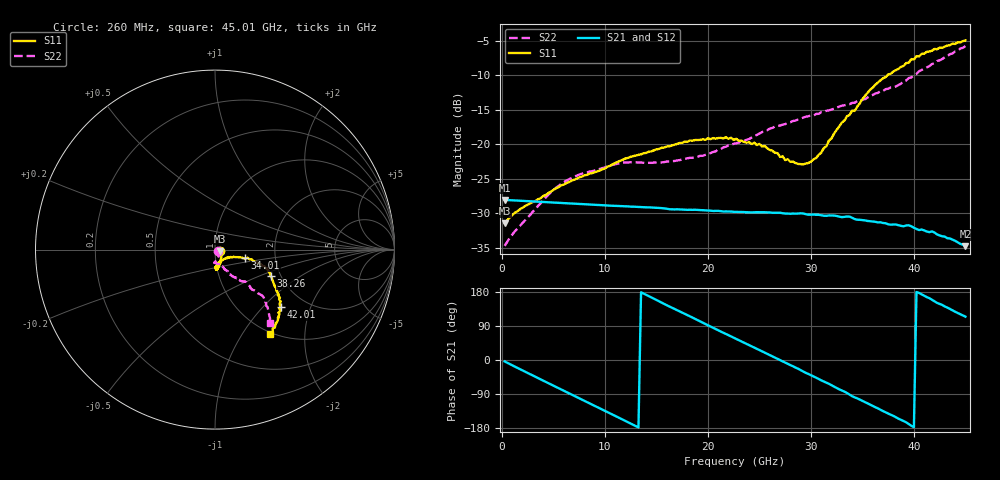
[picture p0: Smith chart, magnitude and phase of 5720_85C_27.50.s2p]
! Device:  ADRF5720
! Description: 0.5dB LSB GaAs MMIC 6-bit Digital Attenuator
! Frequency:  0.000009 -  40 GHz
! Ports:
!	RF1	= Port 1
!	RF2	= Port 2
! Vdd:  3.3 Volt
! Vss:  -3.3 Volt
! Control:  0/3.3 Volt
! State:  27.50 dB attenuation
! Data:  The device was measured using G-S-G Probes on a matrix board.
!  Data was collected using an calibrated 4 port network analyzer.
!  The reference plane for this measurement is at the launchers.
! Note:  Analog Devices supplies this data as a sample of measured data
!  for this product.  Your particular data for this product may vary.
!  Data was taken at 85 degrees C.
!  Analog Devices reserves the right to change this data at anytime.
# GHZ S DB R 45.0
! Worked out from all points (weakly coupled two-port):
!   180 points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, 260 MHz to 45.01 GHz, reference 45 ohm
!   highest |S21| = -28.07 dB at 260 MHz (marker M1); lowest = -34.8 dB at 45.01 GHz (marker M2)
!   lowest |S11| = -31.5 dB at 260 MHz (marker M3), VSWR 1.05, Z = 47.3 - j0.764 ohm
!   |S11| at or under -10 dB: start of sweep to 37.46 GHz
!   |S22| runs from -34.7 to -5.8 dB; largest |S21 - S12| = 0.00027
!   S11 on the Smith chart (normalised r, x): 260 MHz: 1.05, -0.02; 34.01 GHz: 1.40, -0.14; 38.26 GHz: 1.77, -0.59; 42.01 GHz: 1.52, -1.28; 45.01 GHz: 0.97, -1.34
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0.26  -31.47 -17.6  -28.07 -3.7  -28.06 -3.7  -34.73 -26.4
1.26  -29.93 -3.5  -28.15 -17.6  -28.14 -17.5  -32.61 -13.7
4.76  -26.87 -37.6  -28.43 -64.5  -28.41 -64.5  -26.96 -65.6
6.26  -25.63 -46.4  -28.55 -84.5  -28.53 -84.4  -25.28 -75.1
7.76  -24.72 -53.3  -28.67 -104.4  -28.66 -104.4  -24.28 -81.6
11.51  -22.39 -67.5  -28.97 -154.4  -28.96 -154.3  -22.72 -92.2
15.26  -20.69 -75.5  -29.24 154.8  -29.22 154.9  -22.64 -90.0
18.26  -19.46 -81.1  -29.50 115.2  -29.49 115.4  -21.98 -81.7
22.76  -19.22 -86.7  -29.80 55.5  -29.78 55.7  -19.87 -67.5
25.51  -20.24 -85.5  -29.86 19.6  -29.84 19.8  -18.05 -63.7
27.51  -22.31 -78.3  -30.05 -7.0  -30.03 -6.7  -17.10 -59.6
28.76  -22.87 -61.7  -30.05 -23.0  -30.02 -22.7  -16.44 -59.9
30.26  -22.21 -41.2  -30.19 -43.2  -30.17 -43.0  -15.86 -58.7
31.51  -20.31 -24.8  -30.38 -59.7  -30.37 -59.4  -15.17 -57.2
34.01  -15.15 -16.1  -30.66 -95.5  -30.63 -95.4  -14.03 -53.2
34.26  -15.20 -17.4  -30.85 -98.7  -30.85 -98.4  -14.01 -52.4
36.26  -11.40 -17.8  -31.24 -124.6  -31.23 -124.2  -12.68 -49.9
37.76  -9.81 -22.1  -31.66 -144.4  -31.64 -143.9  -11.80 -46.3
38.26  -9.30 -25.3  -31.63 -151.2  -31.62 -150.8  -11.66 -46.1
40.26  -7.26 -35.1  -32.28 179.3  -32.27 179.6  -9.83 -45.6
42.01  -6.21 -41.1  -32.80 154.8  -32.75 155.2  -8.27 -44.9
45.01  -4.99 -57.1  -34.77 114.5  -34.71 114.7  -5.82 -53.3
